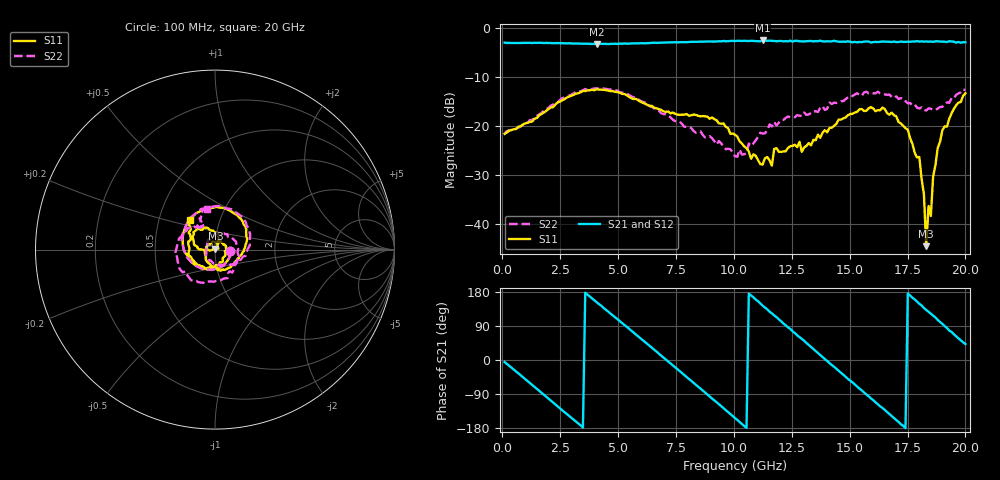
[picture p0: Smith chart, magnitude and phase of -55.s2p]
!Agilent Technologies,N5230C,MY49001569,A.09.33.09
!Agilent N5230C: A.09.33.09
!Date: Monday, July 27, 2015 12:40:56
!Correction: S11(Full 2 Port(1,2))
!S21(Full 2 Port(1,2))
!S12(Full 2 Port(1,2))
!S22(Full 2 Port(1,2))
!S2P File: Measurements: S11, S21, S12, S22:
# Hz S  dB  R 50
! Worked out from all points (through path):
!   201 points, 100 MHz to 20 GHz, reference 50 ohm
!   highest |S21| = -2.49 dB at 11.24 GHz (marker M1); lowest = -3.2 dB at 4.08 GHz (marker M2)
!   group delay of S21, straight-line fit = 144 ps
!   lowest |S11| = -44.6 dB at 18.31 GHz (marker M3), VSWR 1.01, Z = 50.2 + j0.557 ohm
!   |S11| at or under -10 dB: start of sweep to end of sweep
!   |S22| runs from -26.3 to -12.3 dB; largest |S21 - S12| = 0.033
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1e8  -21.60 -6.4  -2.94 -5.4  -2.95 -5.4  -21.49 -5.9
1.7915e9  -17.24 -138.7  -3.01 -91.5  -3.03 -91.6  -16.84 -142.6
3.483e9  -12.81 117.7  -3.17 -177.6  -3.22 -177.9  -12.70 113.9
4.08e9  -12.46 88.9  -3.22 152.5  -3.20 152.4  -12.27 84.2
5.3735e9  -13.67 32.6  -3.15 87.6  -3.14 87.3  -13.39 23.7
6.7665e9  -16.56 -11.1  -2.96 16.5  -2.94 16.2  -16.88 -27.9
7.5625e9  -17.64 -30.6  -2.88 -24.1  -2.88 -24.3  -19.06 -51.8
8.5575e9  -18.01 -55.3  -2.73 -75.4  -2.80 -76.1  -21.06 -79.4
1.005e10  -21.76 -120.4  -2.61 -153.3  -2.64 -153.3  -26.14 -171.0
1.1244e10  -27.88 126.1  -2.49 143.4  -2.66 143.7  -21.52 86.2
1.2239e10  -25.15 29.7  -2.63 91.6  -2.54 91.9  -18.33 23.8
1.3433e10  -22.81 -52.2  -2.68 29.2  -2.63 29.0  -16.96 -30.7
1.43285e10  -19.96 -105.1  -2.57 -17.9  -2.71 -18.7  -15.20 -80.1
1.51245e10  -17.50 -151.1  -2.86 -59.1  -2.67 -60.3  -13.86 -120.5
1.67165e10  -17.68 121.7  -2.77 -142.6  -2.79 -143.2  -13.56 163.1
1.801e10  -26.30 73.6  -2.73 148.3  -2.84 148.6  -16.41 126.2
1.8209e10  -33.93 16.1  -2.74 137.2  -2.79 137.5  -16.69 118.6
1.83085e10  -44.56 69.6  -2.69 132.3  -2.70 131.8  -16.81 119.3
1.8408e10  -36.35 129.6  -2.74 127.1  -2.63 126.8  -16.39 121.0
1.85075e10  -38.39 -174.7  -2.71 122.1  -2.64 120.8  -16.45 124.4
1.8806e10  -24.41 -175.3  -2.65 105.7  -2.75 104.7  -16.44 115.7
2e10  -13.29 130.0  -2.88 42.0  -2.89 40.2  -12.65 101.6
